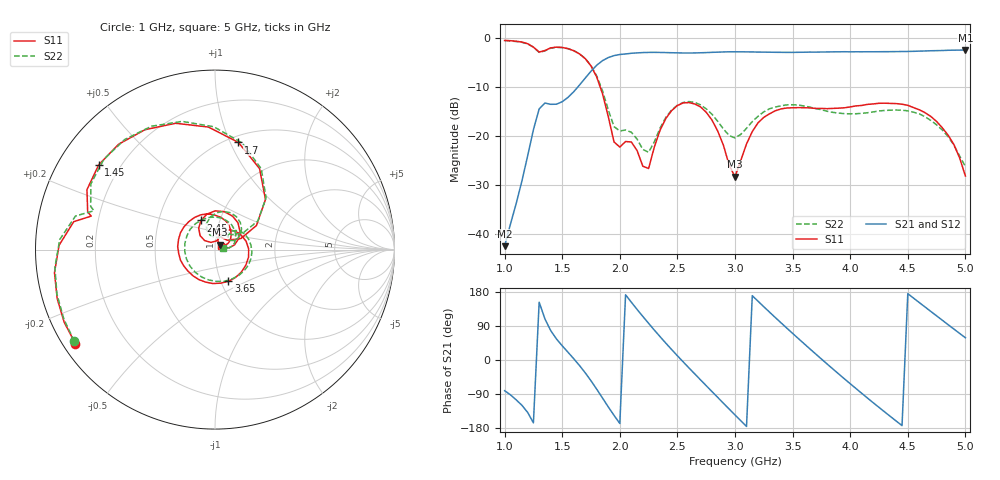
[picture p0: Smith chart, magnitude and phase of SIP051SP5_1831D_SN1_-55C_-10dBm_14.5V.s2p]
# GHz  S  dB  R  50
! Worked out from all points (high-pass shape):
!   81 points, 1 GHz to 5 GHz, reference 50 ohm
!   highest |S21| = -2.50 dB at 5 GHz (marker M1); lowest = -42.6 dB at 1 GHz (marker M2)
!   |S21| within 3 dB of the highest: 1.806 GHz to end of sweep
!   lowest |S11| = -28.4 dB at 3 GHz (marker M3), VSWR 1.08, Z = 52.5 + j2.98 ohm
!   |S11| at or under -10 dB: 1.829 GHz to end of sweep
!   |S22| runs from -26.3 to -0.6 dB; largest |S21 - S12| = 0.0021
!   S11 on the Smith chart (normalised r, x): 1 GHz: 0.04, -0.30; 1.45 GHz: 0.12, +0.32; 1.7 GHz: 0.56, +1.07; 2.45 GHz: 0.81, +0.27; 3.65 GHz: 1.08, -0.40; 5 GHz: 1.07, +0.04
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1  -0.56 -146.1  -42.59 -81.0  -42.13 -82.5  -0.58 -146.9
1.3  -2.92 164.9  -14.54 152.5  -14.51 152.5  -2.99 162.2
1.45  -1.92 143.9  -13.58 55.6  -13.57 55.7  -1.96 141.0
1.7  -4.28 77.7  -8.24 -33.9  -8.24 -33.8  -4.25 75.6
1.85  -11.46 30.2  -4.68 -100.5  -4.68 -100.6  -10.85 33.7
1.95  -21.30 37.3  -3.65 -146.2  -3.68 -146.1  -18.17 42.1
2.05  -21.21 77.1  -3.31 172.1  -3.30 172.1  -18.85 62.8
2.25  -26.71 119.4  -3.00 96.7  -3.00 96.7  -23.40 91.3
2.35  -18.87 136.9  -3.00 61.4  -3.00 61.4  -18.43 112.6
2.45  -14.89 115.7  -3.06 27.6  -3.07 27.5  -14.77 98.4
2.6  -13.25 76.2  -3.12 -20.8  -3.12 -20.8  -13.04 67.0
2.75  -15.22 36.9  -3.04 -67.8  -3.03 -67.7  -14.53 38.0
3  -28.42 48.4  -2.87 -145.0  -2.87 -145.1  -20.47 40.3
3.15  -19.17 65.5  -2.90 169.8  -2.91 169.9  -17.13 47.9
3.35  -14.92 14.9  -2.98 112.1  -2.98 112.1  -14.16 17.6
3.65  -14.34 -67.1  -2.94 29.4  -2.95 29.5  -14.17 -47.4
3.7  -14.45 -80.5  -2.94 16.0  -2.93 16.0  -14.47 -60.6
4.05  -13.93 -163.2  -2.87 -75.2  -2.87 -75.2  -15.53 -161.5
4.35  -13.41 133.3  -2.85 -149.3  -2.86 -149.3  -14.81 114.7
4.6  -14.72 80.7  -2.74 151.6  -2.74 151.5  -15.55 56.5
4.8  -18.41 41.3  -2.62 104.9  -2.61 104.9  -18.86 18.2
5  -28.25 28.9  -2.50 58.6  -2.50 58.6  -26.34 13.5
